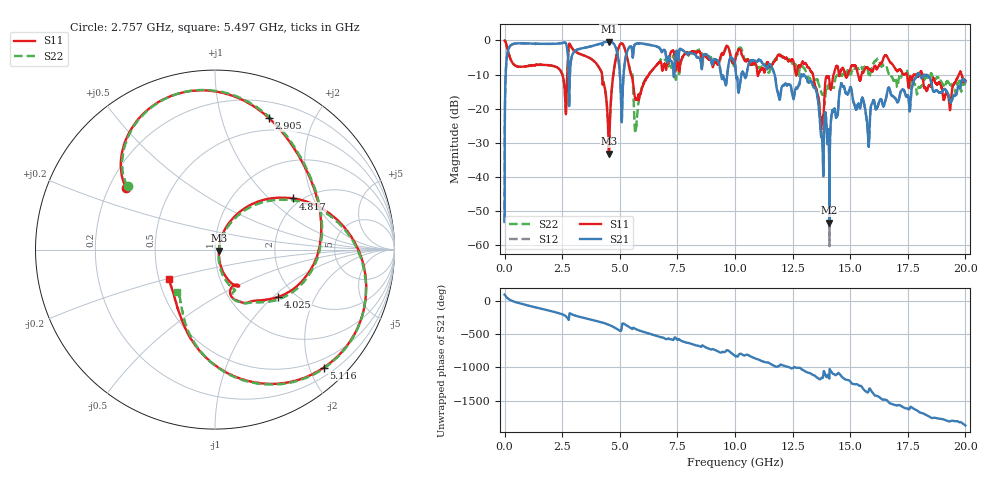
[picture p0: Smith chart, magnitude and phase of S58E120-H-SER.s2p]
!{S58E120}
!Johanson Technology Inc.
!www.johansontechnology.com
!Test Board Conditions:
!Substrate Type  RO4350B
!Substrate Thickness  60 mil
!Substrate Dk  3.66
!TL Type: GCPW
!TL Trace Width  115 mil
!TL Gap  52 mil
!Electrode orientation  Horizontal
!DUT TOPOLOGY	SERIES
!Mounting Pad LxW  55x428 mil
! Created Wed Apr 14 11:02:55 2021
# mhz S ma R 50
! 2 Port Network Data from SP1.SP block
! freq  magS11  angS11  magS21  angS21  magS12  angS12  magS22  angS22
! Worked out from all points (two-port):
!   20001 points, 300 kHz to 20 GHz, reference 50 ohm
!   highest |S21| = -0.31 dB at 4.517 GHz (marker M1); lowest = -53.4 dB at 14.1 GHz (marker M2)
!   |S21| within 3 dB of the highest: 137.9 MHz to 2.737 GHz (2.599 GHz wide, 181 % of centre); 3.018 GHz to 4.881 GHz (1.863 GHz wide, 47.2 % of centre)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
!   lowest |S11| = -33.2 dB at 4.525 GHz (marker M3), VSWR 1.04, Z = 52.2 - j0.547 ohm
!   |S11| at or under -10 dB: 5.486 GHz to 6.263 GHz (777.3 MHz wide, 13.2 % of centre); 13.38 GHz to 14.28 GHz (894.6 MHz wide, 6.47 % of centre); 18.13 GHz to 19.72 GHz (1.591 GHz wide, 8.41 % of centre)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
!   |S22| runs from -33.1 to 0.0 dB; largest |S21 - S12| = 0.012
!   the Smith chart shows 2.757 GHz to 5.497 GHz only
!   S11 on the Smith chart (normalised r, x): 2.757 GHz: 0.27, +0.29; 2.905 GHz: 0.36, +1.43; 4.025 GHz: 1.65, -1.08; 4.817 GHz: 1.82, +1.42; 5.116 GHz: 0.34, -2.24; 5.497 GHz: 0.56, -0.20
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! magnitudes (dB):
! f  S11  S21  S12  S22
! 300 kHz  0.0  -53.2  -53.2  0.0
! 107.3 MHz  -2.0  -4.4  -4.4  -2.0
! 252.3 MHz  -5.4  -1.5  -1.5  -5.4
! 2.757 GHz  -4.4  -5.0  -5.0  -4.4
! 2.905 GHz  -2.0  -5.0  -5.0  -2.0
! 3.334 GHz  -4.1  -2.3  -2.3  -4.1
! 4.025 GHz  -7.1  -1.2  -1.2  -7.1
! 4.517 GHz  -31.8  -0.3  -0.3  -31.1
! 4.525 GHz  -33.2  -0.3  -0.3  -32.8
! 4.817 GHz  -5.7  -1.9  -1.9  -5.7
! 5.116 GHz  -1.0  -16.8  -16.8  -1.0
! 5.497 GHz  -10.3  -1.8  -1.8  -10.0
! 5.709 GHz  -17.2  -1.0  -1.0  -25.1
! 6.667 GHz  -6.7  -2.0  -1.9  -6.8
! 10 GHz  -6.3  -6.9  -6.9  -7.1
! 13.33 GHz  -9.4  -12.2  -12.4  -12.9
! 13.77 GHz  -24.3  -28.3  -27.0  -15.6
! 14.1 GHz  -11.9  -53.4  -60.3  -12.6
! 14.64 GHz  -8.3  -12.9  -12.8  -10.2
! 15.77 GHz  -8.1  -27.9  -27.6  -9.0
! 16.67 GHz  -5.6  -13.8  -13.8  -9.6
! 20 GHz  -11.8  -12.3  -12.2  -13.5
